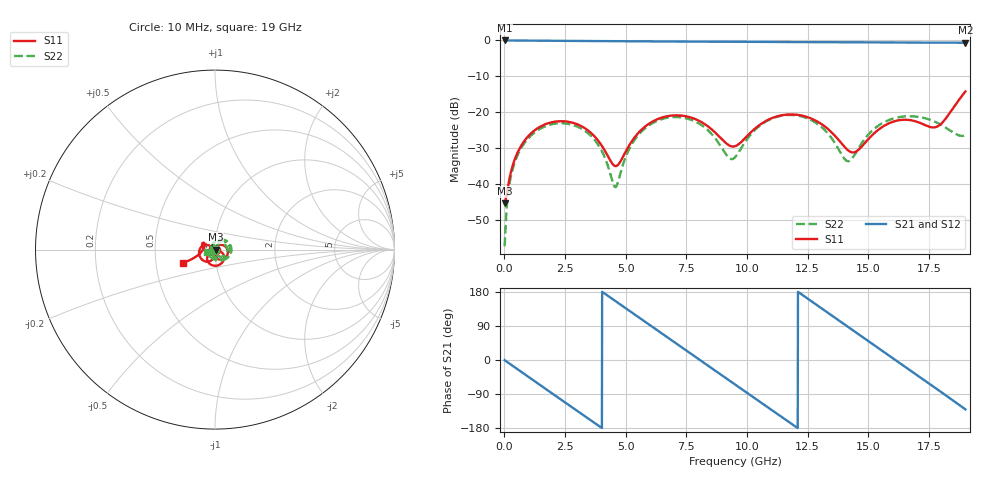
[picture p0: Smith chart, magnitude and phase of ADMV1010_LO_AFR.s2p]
! Analog Devices, Inc.
! 1 Analog Way
! Wilmington, MA 01887
! http://www.analog.com
! Date:  2021-09-07 NN
! Board Name:  ADMV1010-EVALZ Revision B with ADMV1010AEZ installed
! File Description:  Automatic Fixture Removal S-Parameters for LO Port connector and board loss de-embedding
! File Generation:  Calibrated Network Analyzer
! Chip Part Number:  ADMV1010
! Chip Description:  GaAs, MMIC, IQ Downconverter
! Chip Frequency:  12.6 to 15.4 GHz
! Chip Package:  LCC, 4.9 x 4.9 x 1 mm
! LO Port:  ADMV1010AEZ removed and end of trace left open
! Note:
!  Analog Devices supplies this data as a sample of measured data at the evaluation board
!  ports for this product.  Your particular data for this product may vary.
!  Analog Devices reserves the right to change this data at anytime.
!  All lines below in this file are as is from the Network Analyzer.
!Agilent Technologies,N5245A,MY52451809,A.10.47.06
!Automatic Fixture Removal (AFR)
!Date: Friday, August 27, 2021 10:46:59 PM
!S2P File: Measurements: S11,S21,S12,S22:
# MHz S  RI  R 50
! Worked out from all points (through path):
!   1900 points, 10 MHz to 19 GHz, reference 50 ohm
!   highest |S21| = 0.00 dB at 10 MHz (marker M1); lowest = -0.6 dB at 19 GHz (marker M2)
!   group delay of S21, straight-line fit = 124 ps
!   lowest |S11| = -45.5 dB at 10 MHz (marker M3), VSWR 1.01, Z = 50.5 + j0.0464 ohm
!   |S11| at or under -10 dB: start of sweep to end of sweep
!   |S22| runs from -57.4 to -20.8 dB; largest |S21 - S12| = 1.5e-15
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10  0.00531 0.000459  1 -0.00785  1 -0.00785  0.00127 0.000463
280  0.00859 0.0123  0.9748 -0.2176  0.9748 -0.2176  0.00374 0.0126
830  0.0301 0.0264  0.7918 -0.6028  0.7918 -0.6028  0.021 0.0306
2000  0.0715 -0.014  0.00672 -0.9871  0.00672 -0.9871  0.0672 0.0122
3180  0.0293 -0.0564  -0.776 -0.6031  -0.776 -0.6031  0.0461 -0.0364
3930  0.00278 -0.0374  -0.9777 -0.0761  -0.9777 -0.0761  0.00812 -0.0314
4580  0.00994 -0.0146  -0.8899 0.4065  -0.8899 0.4065  -0.00897 -0.000361
5330  0.0392 -0.0172  -0.5155 0.827  -0.5155 0.827  0.00894 0.0383
6340  0.0431 -0.0681  0.2209 0.9431  0.2209 0.9431  0.0678 0.0362
7220  -0.00522 -0.0899  0.7653 0.5879  0.7653 0.5879  0.0834 -0.0167
7960  -0.0401 -0.0664  0.9608 0.0751  0.9608 0.0751  0.0489 -0.0518
8690  -0.0393 -0.034  0.8488 -0.4547  0.8488 -0.4547  -0.000392 -0.0432
9510  -0.0152 -0.0299  0.4084 -0.8698  0.4084 -0.8698  -0.0214 0.00994
10400  -0.0186 -0.059  -0.2403 -0.9258  -0.2403 -0.9258  0.0212 0.0557
11350  -0.0656 -0.0606  -0.7959 -0.5209  -0.7959 -0.5209  0.083 0.0303
12670  -0.0802 0.0107  -0.8546 0.4098  -0.8546 0.4098  0.0559 -0.0526
13490  -0.0439 0.0281  -0.4387 0.8394  -0.4387 0.8394  -0.00148 -0.0431
14210  -0.026 0.0118  0.0792 0.9423  0.0792 0.9423  -0.0204 0.00385
15840  -0.0686 0.0121  0.9167 0.1978  0.9167 0.1978  0.0643 0.0433
16670  -0.0683 0.0374  0.8479 -0.3921  0.8479 -0.3921  0.0877 -0.00419
17600  -0.0578 0.0213  0.3728 -0.8546  0.3728 -0.8546  0.0538 -0.0552
19000  -0.1795 -0.0744  -0.6025 -0.71  -0.6025 -0.71  -0.0455 -0.0139
